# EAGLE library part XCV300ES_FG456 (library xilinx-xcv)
xcv300es_fg456 edit this description Auto generated by make-symbol-device-package-bsdl.ulp Rev. 26 Source: xcv300es_fg456.bsd
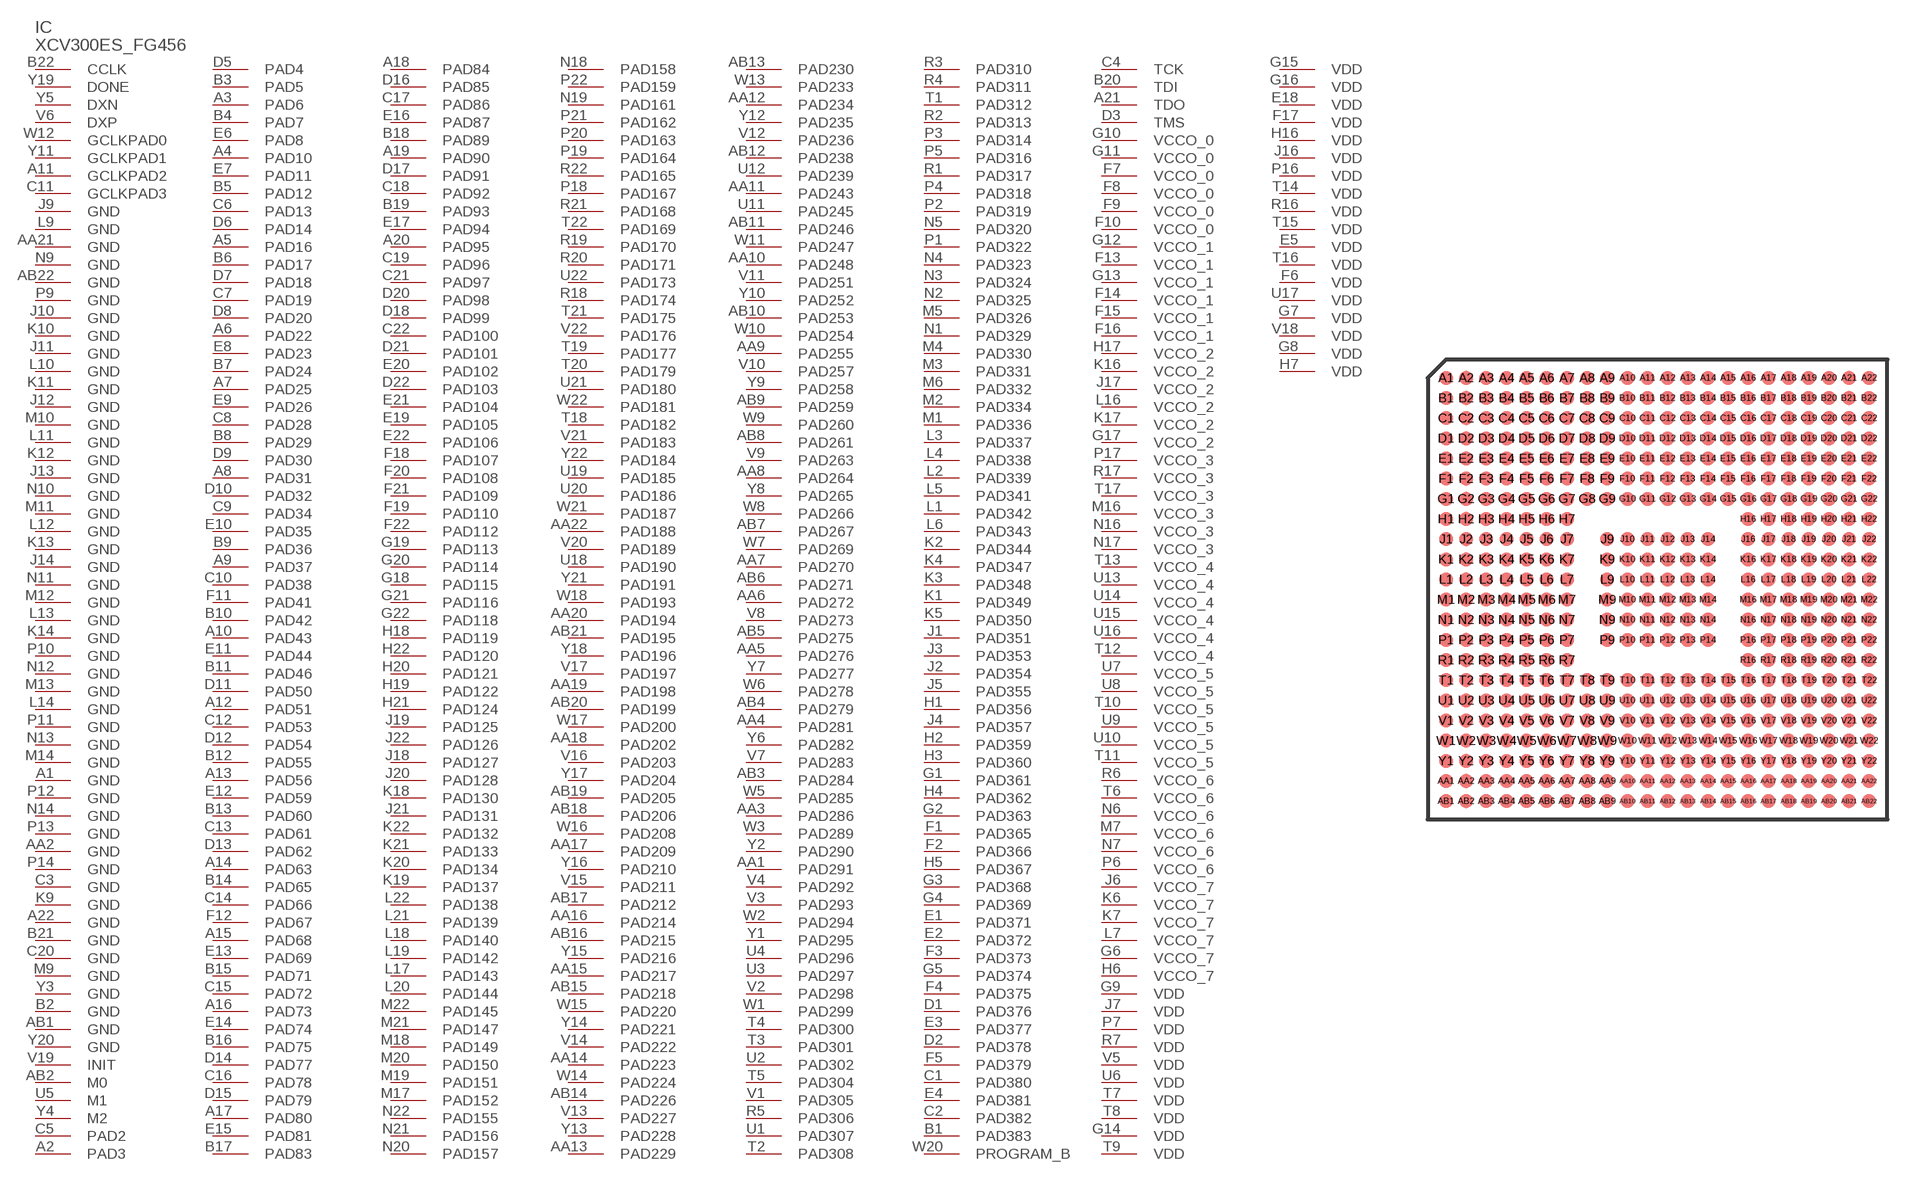
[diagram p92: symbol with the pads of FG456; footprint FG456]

Designator prefix IC

## XCV300ES_FG456 (OC_FARNELL: unknown; OC_NEWARK: unknown)  [FG456]
A1  GND  pwr
A2  PAD3
A3  PAD6
A4  PAD10
A5  PAD16
A6  PAD22
A7  PAD25
A8  PAD31
A9  PAD37
A10  PAD43
A11  GCLKPAD2  in
A12  PAD51
A13  PAD56
A14  PAD63
A15  PAD68
A16  PAD73
A17  PAD80
A18  PAD84
A19  PAD90
A20  PAD95
A21  TDO  out
A22  GND  pwr
AA1  PAD291
AA2  GND  pwr
AA3  PAD286
AA4  PAD281
AA5  PAD276
AA6  PAD272
AA7  PAD270
AA8  PAD264
AA9  PAD255
AA10  PAD248
AA11  PAD243
AA12  PAD234
AA13  PAD229
AA14  PAD223
AA15  PAD217
AA16  PAD214
AA17  PAD209
AA18  PAD202
AA19  PAD198
AA20  PAD194
AA21  GND  pwr
AA22  PAD188
AB1  GND  pwr
AB2  M0  in
AB3  PAD284
AB4  PAD279
AB5  PAD275
AB6  PAD271
AB7  PAD267
AB8  PAD261
AB9  PAD259
AB10  PAD253
AB11  PAD246
AB12  PAD238
AB13  PAD230
AB14  PAD226
AB15  PAD218
AB16  PAD215
AB17  PAD212
AB18  PAD206
AB19  PAD205
AB20  PAD199
AB21  PAD195
AB22  GND  pwr
B1  PAD383
B2  GND  pwr
B3  PAD5
B4  PAD7
B5  PAD12
B6  PAD17
B7  PAD24
B8  PAD29
B9  PAD36
B10  PAD42
B11  PAD46
B12  PAD55
B13  PAD60
B14  PAD65
B15  PAD71
B16  PAD75
B17  PAD83
B18  PAD89
B19  PAD93
B20  TDI  in
B21  GND  pwr
B22  CCLK
C1  PAD380
C2  PAD382
C3  GND  pwr
C4  TCK  in
C5  PAD2
C6  PAD13
C7  PAD19
C8  PAD28
C9  PAD34
C10  PAD38
C11  GCLKPAD3  in
C12  PAD53
C13  PAD61
C14  PAD66
C15  PAD72
C16  PAD78
C17  PAD86
C18  PAD92
C19  PAD96
C20  GND  pwr
C21  PAD97
C22  PAD100
D1  PAD376
D2  PAD378
D3  TMS  in
D5  PAD4
D6  PAD14
D7  PAD18
D8  PAD20
D9  PAD30
D10  PAD32
D11  PAD50
D12  PAD54
D13  PAD62
D14  PAD77
D15  PAD79
D16  PAD85
D17  PAD91
D18  PAD99
D20  PAD98
D21  PAD101
D22  PAD103
E1  PAD371
E2  PAD372
E3  PAD377
E4  PAD381
E5  VDD  pwr
E6  PAD8
E7  PAD11
E8  PAD23
E9  PAD26
E10  PAD35
E11  PAD44
E12  PAD59
E13  PAD69
E14  PAD74
E15  PAD81
E16  PAD87
E17  PAD94
E18  VDD  pwr
E19  PAD105
E20  PAD102
E21  PAD104
E22  PAD106
F1  PAD365
F2  PAD366
F3  PAD373
F4  PAD375
F5  PAD379
F6  VDD  pwr
F7  VCCO_0  pwr
F8  VCCO_0  pwr
F9  VCCO_0  pwr
F10  VCCO_0  pwr
F11  PAD41
F12  PAD67
F13  VCCO_1  pwr
F14  VCCO_1  pwr
F15  VCCO_1  pwr
F16  VCCO_1  pwr
F17  VDD  pwr
F18  PAD107
F19  PAD110
F20  PAD108
F21  PAD109
F22  PAD112
G1  PAD361
G2  PAD363
G3  PAD368
G4  PAD369
G5  PAD374
G6  VCCO_7  pwr
G7  VDD  pwr
G8  VDD  pwr
G9  VDD  pwr
G10  VCCO_0  pwr
G11  VCCO_0  pwr
G12  VCCO_1  pwr
G13  VCCO_1  pwr
G14  VDD  pwr
G15  VDD  pwr
G16  VDD  pwr
G17  VCCO_2  pwr
G18  PAD115
G19  PAD113
G20  PAD114
G21  PAD116
G22  PAD118
H1  PAD356
H2  PAD359
H3  PAD360
H4  PAD362
H5  PAD367
H6  VCCO_7  pwr
H7  VDD  pwr
H16  VDD  pwr
H17  VCCO_2  pwr
H18  PAD119
H19  PAD122
H20  PAD121
H21  PAD124
H22  PAD120
J1  PAD351
J2  PAD354
J3  PAD353
J4  PAD357
J5  PAD355
J6  VCCO_7  pwr
J7  VDD  pwr
J9  GND  pwr
J10  GND  pwr
J11  GND  pwr
J12  GND  pwr
J13  GND  pwr
J14  GND  pwr
J16  VDD  pwr
J17  VCCO_2  pwr
J18  PAD127
J19  PAD125
J20  PAD128
J21  PAD131
J22  PAD126
K1  PAD349
K2  PAD344
K3  PAD348
K4  PAD347
K5  PAD350
K6  VCCO_7  pwr
K7  VCCO_7  pwr
K9  GND  pwr
K10  GND  pwr
K11  GND  pwr
K12  GND  pwr
K13  GND  pwr
K14  GND  pwr
K16  VCCO_2  pwr
K17  VCCO_2  pwr
K18  PAD130
K19  PAD137
K20  PAD134
K21  PAD133
K22  PAD132
L1  PAD342
L2  PAD339
L3  PAD337
L4  PAD338
L5  PAD341
L6  PAD343
L7  VCCO_7  pwr
L9  GND  pwr
L10  GND  pwr
L11  GND  pwr
L12  GND  pwr
L13  GND  pwr
L14  GND  pwr
L16  VCCO_2  pwr
L17  PAD143
L18  PAD140
L19  PAD142
L20  PAD144
L21  PAD139
L22  PAD138
M1  PAD336
M2  PAD334
M3  PAD331
M4  PAD330
M5  PAD326
M6  PAD332
M7  VCCO_6  pwr
M9  GND  pwr
M10  GND  pwr
M11  GND  pwr
M12  GND  pwr
M13  GND  pwr
M14  GND  pwr
M16  VCCO_3  pwr
M17  PAD152
M18  PAD149
M19  PAD151
M20  PAD150
M21  PAD147
M22  PAD145
N1  PAD329
N2  PAD325
N3  PAD324
N4  PAD323
N5  PAD320
N6  VCCO_6  pwr
N7  VCCO_6  pwr
N9  GND  pwr
N10  GND  pwr
N11  GND  pwr
N12  GND  pwr
N13  GND  pwr
N14  GND  pwr
N16  VCCO_3  pwr
N17  VCCO_3  pwr
N18  PAD158
N19  PAD161
N20  PAD157
N21  PAD156
N22  PAD155
P1  PAD322
P2  PAD319
P3  PAD314
P4  PAD318
P5  PAD316
P6  VCCO_6  pwr
P7  VDD  pwr
P9  GND  pwr
P10  GND  pwr
P11  GND  pwr
P12  GND  pwr
P13  GND  pwr
P14  GND  pwr
P16  VDD  pwr
P17  VCCO_3  pwr
P18  PAD167
P19  PAD164
P20  PAD163
P21  PAD162
P22  PAD159
R1  PAD317
R2  PAD313
R3  PAD310
R4  PAD311
R5  PAD306
R6  VCCO_6  pwr
R7  VDD  pwr
R16  VDD  pwr
R17  VCCO_3  pwr
R18  PAD174
R19  PAD170
R20  PAD171
R21  PAD168
R22  PAD165
T1  PAD312
T2  PAD308
T3  PAD301
T4  PAD300
T5  PAD304
T6  VCCO_6  pwr
T7  VDD  pwr
T8  VDD  pwr
T9  VDD  pwr
T10  VCCO_5  pwr
T11  VCCO_5  pwr
T12  VCCO_4  pwr
T13  VCCO_4  pwr
T14  VDD  pwr
T15  VDD  pwr
T16  VDD  pwr
T17  VCCO_3  pwr
T18  PAD182
T19  PAD177
T20  PAD179
T21  PAD175
T22  PAD169
U1  PAD307
U2  PAD302
U3  PAD297
U4  PAD296
U5  M1  in
U6  VDD  pwr
U7  VCCO_5  pwr
U8  VCCO_5  pwr
U9  VCCO_5  pwr
U10  VCCO_5  pwr
U11  PAD245
U12  PAD239
U13  VCCO_4  pwr
U14  VCCO_4  pwr
U15  VCCO_4  pwr
U16  VCCO_4  pwr
U17  VDD  pwr
U18  PAD190
U19  PAD185
U20  PAD186
U21  PAD180
U22  PAD173
V1  PAD305
V2  PAD298
V3  PAD293
V4  PAD292
V5  VDD  pwr
V6  DXP  pas
V7  PAD283
V8  PAD273
V9  PAD263
V10  PAD257
V11  PAD251
V12  PAD236
V13  PAD227
V14  PAD222
V15  PAD211
V16  PAD203
V17  PAD197
V18  VDD  pwr
V19  INIT
V20  PAD189
V21  PAD183
V22  PAD176
W1  PAD299
W2  PAD294
W3  PAD289
W5  PAD285
W6  PAD278
W7  PAD269
W8  PAD266
W9  PAD260
W10  PAD254
W11  PAD247
W12  GCLKPAD0  in
W13  PAD233
W14  PAD224
W15  PAD220
W16  PAD208
W17  PAD200
W18  PAD193
W20  PROGRAM_B  in
W21  PAD187
W22  PAD181
Y1  PAD295
Y2  PAD290
Y3  GND  pwr
Y4  M2  in
Y5  DXN  pas
Y6  PAD282
Y7  PAD277
Y8  PAD265
Y9  PAD258
Y10  PAD252
Y11  GCLKPAD1  in
Y12  PAD235
Y13  PAD228
Y14  PAD221
Y15  PAD216
Y16  PAD210
Y17  PAD204
Y18  PAD196
Y19  DONE
Y20  GND  pwr
Y21  PAD191
Y22  PAD184

## Footprint FG456 (pad centres in mm)
xcv150_fg456 edit this description Auto generated by make-symbol-device-package-bsdl.ulp Rev. 26 Source: xcv150_fg456.bsd
smd 0.7 x 0.7: A1 -10.5,10.5; A2 -9.5,10.5; A3 -8.5,10.5; A4 -7.5,10.5; A5 -6.5,10.5; A6 -5.5,10.5; A7 -4.5,10.5; A8 -3.5,10.5; A9 -2.5,10.5; A10 -1.5,10.5; A11 -0.5,10.5; A12 0.5,10.5; A13 1.5,10.5; A14 2.5,10.5; A15 3.5,10.5; A16 4.5,10.5; A17 5.5,10.5; A18 6.5,10.5; A19 7.5,10.5; A20 8.5,10.5; A21 9.5,10.5; A22 10.5,10.5; AA1 -10.5,-9.5; AA2 -9.5,-9.5; AA3 -8.5,-9.5; AA4 -7.5,-9.5; AA5 -6.5,-9.5; AA6 -5.5,-9.5; AA7 -4.5,-9.5; AA8 -3.5,-9.5; AA9 -2.5,-9.5; AA10 -1.5,-9.5; AA11 -0.5,-9.5; AA12 0.5,-9.5; AA13 1.5,-9.5; AA14 2.5,-9.5; AA15 3.5,-9.5; AA16 4.5,-9.5; AA17 5.5,-9.5; AA18 6.5,-9.5; AA19 7.5,-9.5; AA20 8.5,-9.5; AA21 9.5,-9.5; AA22 10.5,-9.5; AB1 -10.5,-10.5; AB2 -9.5,-10.5; AB3 -8.5,-10.5; AB4 -7.5,-10.5; AB5 -6.5,-10.5; AB6 -5.5,-10.5; AB7 -4.5,-10.5; AB8 -3.5,-10.5; AB9 -2.5,-10.5; AB10 -1.5,-10.5; AB11 -0.5,-10.5; AB12 0.5,-10.5; AB13 1.5,-10.5; AB14 2.5,-10.5; AB15 3.5,-10.5; AB16 4.5,-10.5; AB17 5.5,-10.5; AB18 6.5,-10.5; AB19 7.5,-10.5; AB20 8.5,-10.5; AB21 9.5,-10.5; AB22 10.5,-10.5; B1 -10.5,9.5; B2 -9.5,9.5; B3 -8.5,9.5; B4 -7.5,9.5; B5 -6.5,9.5; B6 -5.5,9.5; B7 -4.5,9.5; B8 -3.5,9.5; B9 -2.5,9.5; B10 -1.5,9.5; B11 -0.5,9.5; B12 0.5,9.5; B13 1.5,9.5; B14 2.5,9.5; B15 3.5,9.5; B16 4.5,9.5; B17 5.5,9.5; B18 6.5,9.5; B19 7.5,9.5; B20 8.5,9.5; B21 9.5,9.5; B22 10.5,9.5; C1 -10.5,8.5; C2 -9.5,8.5; C3 -8.5,8.5; C4 -7.5,8.5; C5 -6.5,8.5; C6 -5.5,8.5; C7 -4.5,8.5; C8 -3.5,8.5; C9 -2.5,8.5; C10 -1.5,8.5; C11 -0.5,8.5; C12 0.5,8.5; C13 1.5,8.5; C14 2.5,8.5; C15 3.5,8.5; C16 4.5,8.5; C17 5.5,8.5; C18 6.5,8.5; C19 7.5,8.5; C20 8.5,8.5; C21 9.5,8.5; C22 10.5,8.5; D1 -10.5,7.5; D2 -9.5,7.5; D3 -8.5,7.5; D4 -7.5,7.5; D5 -6.5,7.5; D6 -5.5,7.5; D7 -4.5,7.5; D8 -3.5,7.5; D9 -2.5,7.5; D10 -1.5,7.5; D11 -0.5,7.5; D12 0.5,7.5; D13 1.5,7.5; D14 2.5,7.5; D15 3.5,7.5; D16 4.5,7.5; D17 5.5,7.5; D18 6.5,7.5; D19 7.5,7.5; D20 8.5,7.5; D21 9.5,7.5; D22 10.5,7.5; E1 -10.5,6.5; E2 -9.5,6.5; E3 -8.5,6.5; E4 -7.5,6.5; E5 -6.5,6.5; E6 -5.5,6.5; E7 -4.5,6.5; E8 -3.5,6.5; E9 -2.5,6.5; E10 -1.5,6.5; E11 -0.5,6.5; E12 0.5,6.5; E13 1.5,6.5; E14 2.5,6.5; E15 3.5,6.5; E16 4.5,6.5; E17 5.5,6.5; E18 6.5,6.5; E19 7.5,6.5; E20 8.5,6.5; E21 9.5,6.5; E22 10.5,6.5; F1 -10.5,5.5; F2 -9.5,5.5; F3 -8.5,5.5; F4 -7.5,5.5; F5 -6.5,5.5; F6 -5.5,5.5; F7 -4.5,5.5; F8 -3.5,5.5; F9 -2.5,5.5; F10 -1.5,5.5; F11 -0.5,5.5; F12 0.5,5.5; F13 1.5,5.5; F14 2.5,5.5; F15 3.5,5.5; F16 4.5,5.5; F17 5.5,5.5; F18 6.5,5.5; F19 7.5,5.5; F20 8.5,5.5; F21 9.5,5.5; F22 10.5,5.5; G1 -10.5,4.5; G2 -9.5,4.5; G3 -8.5,4.5; G4 -7.5,4.5; G5 -6.5,4.5; G6 -5.5,4.5; G7 -4.5,4.5; G8 -3.5,4.5; G9 -2.5,4.5; G10 -1.5,4.5; G11 -0.5,4.5; G12 0.5,4.5; G13 1.5,4.5; G14 2.5,4.5; G15 3.5,4.5; G16 4.5,4.5; G17 5.5,4.5; G18 6.5,4.5; G19 7.5,4.5; G20 8.5,4.5; G21 9.5,4.5; G22 10.5,4.5; H1 -10.5,3.5; H2 -9.5,3.5; H3 -8.5,3.5; H4 -7.5,3.5; H5 -6.5,3.5; H6 -5.5,3.5; H7 -4.5,3.5; H16 4.5,3.5; H17 5.5,3.5; H18 6.5,3.5; H19 7.5,3.5; H20 8.5,3.5; H21 9.5,3.5; H22 10.5,3.5; J1 -10.5,2.5; J2 -9.5,2.5; J3 -8.5,2.5; J4 -7.5,2.5; J5 -6.5,2.5; J6 -5.5,2.5; J7 -4.5,2.5; J9 -2.5,2.5; J10 -1.5,2.5; J11 -0.5,2.5; J12 0.5,2.5; J13 1.5,2.5; J14 2.5,2.5; J16 4.5,2.5; J17 5.5,2.5; J18 6.5,2.5; J19 7.5,2.5; J20 8.5,2.5; J21 9.5,2.5; J22 10.5,2.5; K1 -10.5,1.5; K2 -9.5,1.5; K3 -8.5,1.5; K4 -7.5,1.5; K5 -6.5,1.5; K6 -5.5,1.5; K7 -4.5,1.5; K9 -2.5,1.5; K10 -1.5,1.5; K11 -0.5,1.5; K12 0.5,1.5; K13 1.5,1.5; K14 2.5,1.5; K16 4.5,1.5; K17 5.5,1.5; K18 6.5,1.5; K19 7.5,1.5; K20 8.5,1.5; K21 9.5,1.5; K22 10.5,1.5; L1 -10.5,0.5; L2 -9.5,0.5; L3 -8.5,0.5; L4 -7.5,0.5; L5 -6.5,0.5; L6 -5.5,0.5; L7 -4.5,0.5; L9 -2.5,0.5; L10 -1.5,0.5; L11 -0.5,0.5; L12 0.5,0.5; L13 1.5,0.5; L14 2.5,0.5; L16 4.5,0.5; L17 5.5,0.5; L18 6.5,0.5; L19 7.5,0.5; L20 8.5,0.5; L21 9.5,0.5; L22 10.5,0.5; M1 -10.5,-0.5; M2 -9.5,-0.5; M3 -8.5,-0.5; M4 -7.5,-0.5; M5 -6.5,-0.5; M6 -5.5,-0.5; M7 -4.5,-0.5; M9 -2.5,-0.5; M10 -1.5,-0.5; M11 -0.5,-0.5; M12 0.5,-0.5; M13 1.5,-0.5; M14 2.5,-0.5; M16 4.5,-0.5; M17 5.5,-0.5; M18 6.5,-0.5; M19 7.5,-0.5; M20 8.5,-0.5; M21 9.5,-0.5; M22 10.5,-0.5; N1 -10.5,-1.5; N2 -9.5,-1.5; N3 -8.5,-1.5; N4 -7.5,-1.5; N5 -6.5,-1.5; N6 -5.5,-1.5; N7 -4.5,-1.5; N9 -2.5,-1.5; N10 -1.5,-1.5; N11 -0.5,-1.5; N12 0.5,-1.5; N13 1.5,-1.5; N14 2.5,-1.5; N16 4.5,-1.5; N17 5.5,-1.5; N18 6.5,-1.5; N19 7.5,-1.5; N20 8.5,-1.5; N21 9.5,-1.5; N22 10.5,-1.5; P1 -10.5,-2.5; P2 -9.5,-2.5; P3 -8.5,-2.5; P4 -7.5,-2.5; P5 -6.5,-2.5; P6 -5.5,-2.5; P7 -4.5,-2.5; P9 -2.5,-2.5; P10 -1.5,-2.5; P11 -0.5,-2.5; P12 0.5,-2.5; P13 1.5,-2.5; P14 2.5,-2.5; P16 4.5,-2.5; P17 5.5,-2.5; P18 6.5,-2.5; P19 7.5,-2.5; P20 8.5,-2.5; P21 9.5,-2.5; P22 10.5,-2.5; R1 -10.5,-3.5; R2 -9.5,-3.5; R3 -8.5,-3.5; R4 -7.5,-3.5; R5 -6.5,-3.5; R6 -5.5,-3.5; R7 -4.5,-3.5; R16 4.5,-3.5; R17 5.5,-3.5; R18 6.5,-3.5; R19 7.5,-3.5; R20 8.5,-3.5; R21 9.5,-3.5; R22 10.5,-3.5; T1 -10.5,-4.5; T2 -9.5,-4.5; T3 -8.5,-4.5; T4 -7.5,-4.5; T5 -6.5,-4.5; T6 -5.5,-4.5; T7 -4.5,-4.5; T8 -3.5,-4.5; T9 -2.5,-4.5; T10 -1.5,-4.5; T11 -0.5,-4.5; T12 0.5,-4.5; T13 1.5,-4.5; T14 2.5,-4.5; T15 3.5,-4.5; T16 4.5,-4.5; T17 5.5,-4.5; T18 6.5,-4.5; T19 7.5,-4.5; T20 8.5,-4.5; T21 9.5,-4.5; T22 10.5,-4.5; U1 -10.5,-5.5; U2 -9.5,-5.5; U3 -8.5,-5.5; U4 -7.5,-5.5; U5 -6.5,-5.5; U6 -5.5,-5.5; U7 -4.5,-5.5; U8 -3.5,-5.5; U9 -2.5,-5.5; U10 -1.5,-5.5; U11 -0.5,-5.5; U12 0.5,-5.5; U13 1.5,-5.5; U14 2.5,-5.5; U15 3.5,-5.5; U16 4.5,-5.5; U17 5.5,-5.5; U18 6.5,-5.5; U19 7.5,-5.5; U20 8.5,-5.5; U21 9.5,-5.5; U22 10.5,-5.5; V1 -10.5,-6.5; V2 -9.5,-6.5; V3 -8.5,-6.5; V4 -7.5,-6.5; V5 -6.5,-6.5; V6 -5.5,-6.5; V7 -4.5,-6.5; V8 -3.5,-6.5; V9 -2.5,-6.5; V10 -1.5,-6.5; V11 -0.5,-6.5; V12 0.5,-6.5; V13 1.5,-6.5; V14 2.5,-6.5; V15 3.5,-6.5; V16 4.5,-6.5; V17 5.5,-6.5; V18 6.5,-6.5; V19 7.5,-6.5; V20 8.5,-6.5; V21 9.5,-6.5; V22 10.5,-6.5; W1 -10.5,-7.5; W2 -9.5,-7.5; W3 -8.5,-7.5; W4 -7.5,-7.5; W5 -6.5,-7.5; W6 -5.5,-7.5; W7 -4.5,-7.5; W8 -3.5,-7.5; W9 -2.5,-7.5; W10 -1.5,-7.5; W11 -0.5,-7.5; W12 0.5,-7.5; W13 1.5,-7.5; W14 2.5,-7.5; W15 3.5,-7.5; W16 4.5,-7.5; W17 5.5,-7.5; W18 6.5,-7.5; W19 7.5,-7.5; W20 8.5,-7.5; W21 9.5,-7.5; W22 10.5,-7.5; Y1 -10.5,-8.5; Y2 -9.5,-8.5; Y3 -8.5,-8.5; Y4 -7.5,-8.5; Y5 -6.5,-8.5; Y6 -5.5,-8.5; Y7 -4.5,-8.5; Y8 -3.5,-8.5; Y9 -2.5,-8.5; Y10 -1.5,-8.5; Y11 -0.5,-8.5; Y12 0.5,-8.5; Y13 1.5,-8.5; Y14 2.5,-8.5; Y15 3.5,-8.5; Y16 4.5,-8.5; Y17 5.5,-8.5; Y18 6.5,-8.5; Y19 7.5,-8.5; Y20 8.5,-8.5; Y21 9.5,-8.5; Y22 10.5,-8.5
